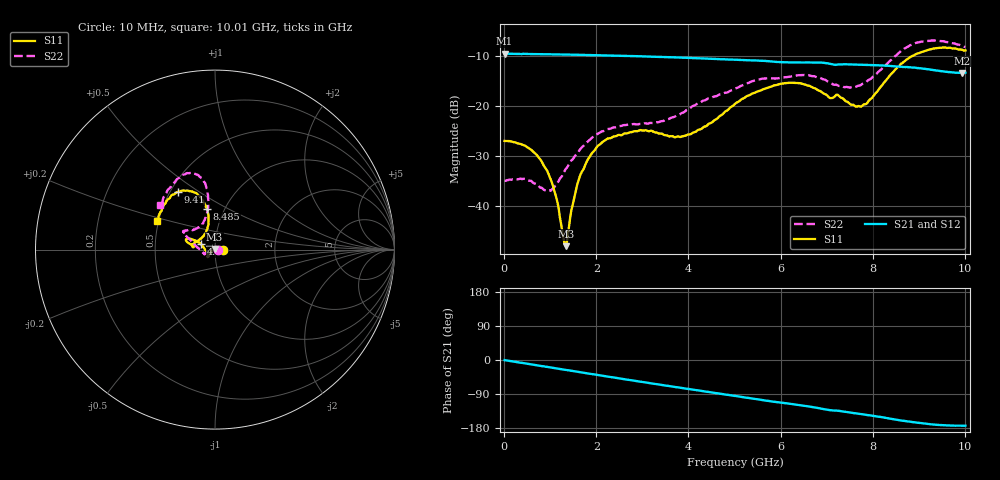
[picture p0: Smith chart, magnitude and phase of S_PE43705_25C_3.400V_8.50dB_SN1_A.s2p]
! Device ID: PE43705
! Serial: 1
! Insertion: A
! Impedance: 50 ohm
! Temp: 25C
! VDD: 3.400V
! Attenuation Step: 8.50dB
#  Hz  S  RI  R  50
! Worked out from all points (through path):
!   401 points, 10 MHz to 10.01 GHz, reference 50 ohm
!   highest |S21| = -9.50 dB at 10 MHz (marker M1); lowest = -13.4 dB at 9.935 GHz (marker M2)
!   group delay of S21, straight-line fit = 50 ps
!   lowest |S11| = -48.1 dB at 1.335 GHz (marker M3), VSWR 1.01, Z = 49.7 + j0.282 ohm
!   |S11| at or under -10 dB: start of sweep to 8.854 GHz
!   |S22| runs from -37.0 to -6.9 dB; largest |S21 - S12| = 0.0031
!   S11 on the Smith chart (normalised r, x): 10 MHz: 1.09, -0.00; 4.76 GHz: 0.85, +0.05; 8.485 GHz: 0.83, +0.40; 9.41 GHz: 0.55, +0.41; 10.01 GHz: 0.49, +0.18
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1e7  0.0447 -2.03e-06  0.3348 -0.00147  0.3351 -0.00147  0.0178 0.00022
4.85e8  0.037 0.0126  0.3277 -0.0564  0.3278 -0.0561  0.0125 0.0133
8.35e8  0.0224 0.0146  0.3171 -0.0942  0.317 -0.0939  0.000242 0.0149
1.085e9  0.0102 0.01  0.306 -0.12  0.306 -0.1199  -0.0111 0.0105
1.285e9  0.000305 0.00486  0.2966 -0.1396  0.2968 -0.1396  -0.0204 0.00618
1.335e9  -0.00273 0.00283  0.2939 -0.1447  0.2941 -0.1445  -0.023 0.00434
1.535e9  -0.0122 -0.00407  0.2824 -0.1636  0.2825 -0.1634  -0.0314 -0.00158
1.685e9  -0.019 -0.0107  0.273 -0.177  0.273 -0.1769  -0.0379 -0.00703
2.21e9  -0.034 -0.0309  0.2351 -0.2193  0.2353 -0.2192  -0.0531 -0.0221
3.36e9  -0.0394 -0.0354  0.1325 -0.2809  0.133 -0.2805  -0.0671 -0.0161
4.01e9  -0.0514 -0.00797  0.0688 -0.2954  0.0691 -0.2951  -0.0929 0.00779
4.76e9  -0.0782 0.0312  -0.00283 -0.2939  -0.00222 -0.2937  -0.1265 0.0442
5.01e9  -0.0955 0.0437  -0.0256 -0.2895  -0.0252 -0.2898  -0.1391 0.055
5.985e9  -0.1547 0.0611  -0.1041 -0.2551  -0.1026 -0.2553  -0.1669 0.0924
6.685e9  -0.1497 0.0373  -0.1531 -0.2257  -0.1532 -0.2256  -0.1693 0.1051
7.71e9  -0.0686 0.0721  -0.2046 -0.159  -0.2041 -0.1594  -0.0692 0.1442
8.36e9  -0.0369 0.196  -0.2277 -0.1094  -0.2268 -0.1105  -0.0377 0.2774
8.485e9  -0.0449 0.2273  -0.2299 -0.0977  -0.229 -0.0993  -0.0417 0.3138
8.91e9  -0.0997 0.3109  -0.2334 -0.0649  -0.2319 -0.065  -0.0934 0.4147
9.41e9  -0.2077 0.3214  -0.2235 -0.0345  -0.2226 -0.0347  -0.1835 0.4152
9.935e9  -0.3136 0.1893  -0.213 -0.0251  -0.2141 -0.0253  -0.291 0.2741
1.001e10  -0.3227 0.1614  -0.2142 -0.0249  -0.2152 -0.0259  -0.3038 0.246
